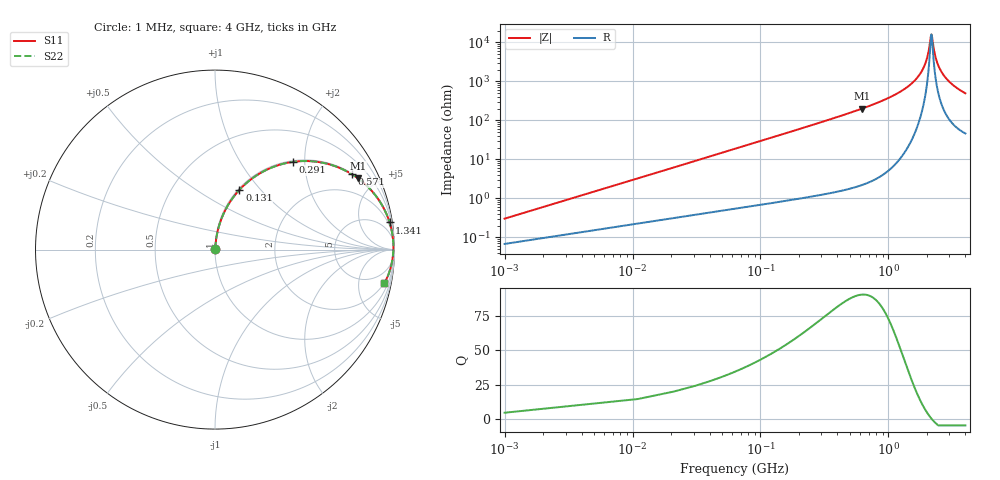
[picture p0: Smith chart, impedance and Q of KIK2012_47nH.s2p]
!version-2
!date-01.2022
!Series
# MHz S RI R 50
!Freq ReS11 ImS11 ReS21 ImS21 ReS12 ImS12 ReS22 ImS22
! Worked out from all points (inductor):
!   401 points, 1 MHz to 4 GHz, reference 50 ohm
!   read as one part in series: L = 47 nH near 21 MHz
!   highest Q = 90.8 at 621 MHz (marker M1), where L = 51.2 nH
!   self-resonance near 2.171 GHz
!   S11 on the Smith chart (normalised r, x): 1 MHz: 1.00, +0.01; 131 MHz: 1.02, +0.78; 291 MHz: 1.02, +1.75; 571 MHz: 1.04, +3.62; 1.341 GHz: 1, +13; 4 GHz: 2, -10
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1  0.000691 0.00295  0.9993 -0.00295  0.9993 -0.00295  0.000691 0.00295
31  0.012 0.0901  0.988 -0.0901  0.988 -0.0901  0.012 0.0901
41  0.0186 0.1183  0.9814 -0.1183  0.9814 -0.1183  0.0186 0.1183
81  0.0594 0.2239  0.9406 -0.2239  0.9406 -0.2239  0.0594 0.2239
131  0.136 0.3328  0.864 -0.3328  0.864 -0.3328  0.136 0.3328
201  0.2673 0.4344  0.7327 -0.4344  0.7327 -0.4344  0.2673 0.4344
291  0.4346 0.4888  0.5654 -0.4888  0.5654 -0.4888  0.4346 0.4888
571  0.764 0.4191  0.236 -0.4191  0.236 -0.4191  0.764 0.4191
621  0.797 0.3968  0.203 -0.3968  0.203 -0.3968  0.797 0.3968
671  0.8249 0.3746  0.1751 -0.3746  0.1751 -0.3746  0.8249 0.3746
1341  0.9728 0.1513  0.0272 -0.1513  0.0272 -0.1513  0.9728 0.1513
1761  0.9911 0.0648  0.00891 -0.0648  0.00891 -0.0648  0.9911 0.0648
2001  0.9938 0.0252  0.00617 -0.0252  0.00617 -0.0252  0.9938 0.0252
2071  0.994 0.0145  0.00603 -0.0145  0.00603 -0.0145  0.994 0.0145
2151  0.9938 0.00287  0.00617 -0.00287  0.00617 -0.00287  0.9938 0.00287
2171  0.9937 1.98e-05  0.00625 -1.98e-05  0.00625 -1.98e-05  0.9937 1.98e-05
2291  0.9929 -0.0165  0.00709 0.0165  0.00709 0.0165  0.9929 -0.0165
2371  0.9921 -0.027  0.00794 0.027  0.00794 0.027  0.9921 -0.027
2501  0.9902 -0.0434  0.00979 0.0434  0.00979 0.0434  0.9902 -0.0434
2671  0.9871 -0.0636  0.0129 0.0636  0.0129 0.0636  0.9871 -0.0636
3341  0.9687 -0.1321  0.0313 0.1321  0.0313 0.1321  0.9687 -0.1321
4000  0.9443 -0.187  0.0557 0.187  0.0557 0.187  0.9443 -0.187
